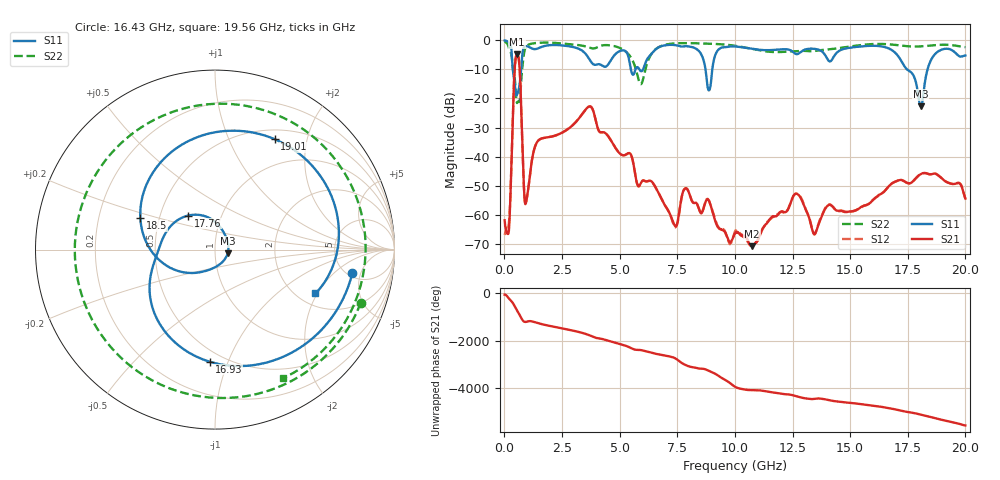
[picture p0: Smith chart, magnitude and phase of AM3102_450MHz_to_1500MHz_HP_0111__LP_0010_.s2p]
!Agilent Technologies,E8364B,MY43040894,A.07.50.67
!Agilent E8364B: A.07.50.67
!Date: Thursday, January 11, 2018 05:51:23
!Correction: S11(Full 2 Port(1,2))
!S21(Full 2 Port(1,2))
!S12(Full 2 Port(1,2))
!S22(Full 2 Port(1,2))
!S2P File: Measurements: S11, S21, S12, S22:
# Hz S  dB  R 50
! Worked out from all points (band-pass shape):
!   1601 points, 10 MHz to 20 GHz, reference 50 ohm
!   highest |S21| = -4.89 dB at 547.2 MHz (marker M1); lowest = -70.8 dB at 10.74 GHz (marker M2)
!   |S21| within 3 dB of the highest: 466.6 MHz to 646 MHz (179.3 MHz wide, 32.2 % of centre)
!   lowest |S11| = -22.7 dB at 18.06 GHz (marker M3), VSWR 1.16, Z = 57.5 - j2.39 ohm
!   |S11| at or under -10 dB: 366.7 MHz to 727.4 MHz (360.6 MHz wide, 65.9 % of centre); 8.724 GHz to 9.02 GHz (295.9 MHz wide, 3.33 % of centre); 17.47 GHz to 18.36 GHz (890.2 MHz wide, 4.97 % of centre)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
!   |S22| runs from -21.6 to -0.4 dB; largest |S21 - S12| = 0.0011
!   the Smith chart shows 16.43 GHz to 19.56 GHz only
!   S11 on the Smith chart (normalised r, x): 16.43 GHz: 5.55, -3.61; 16.93 GHz: 0.42, -0.86; 17.76 GHz: 0.70, +0.28; 18.5 GHz: 0.39, +0.17; 19.01 GHz: 0.62, +1.49; 19.56 GHz: 2.47, -1.92
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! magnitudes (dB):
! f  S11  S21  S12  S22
! 10 MHz  -0.1  -61.9  -66.9  -0.4
! 197.4 MHz  -0.7  -65.4  -62.9  -2.7
! 547.2 MHz  -18.5  -4.9  -4.9  -21.6
! 947 MHz  -2.0  -55.5  -55.4  -2.1
! 1.434 GHz  -2.9  -34.8  -34.9  -0.9
! 3.346 GHz  -3.4  -25.7  -25.7  -1.8
! 5.92 GHz  -10.6  -49.1  -49.2  -15.1
! 6.682 GHz  -2.5  -52.4  -52.4  -2.4
! 8.881 GHz  -17.2  -55.3  -55.2  -1.2
! 10.01 GHz  -2.1  -66.4  -65.7  -1.9
! 10.74 GHz  -2.9  -70.8  -70.5  -3.0
! 12.64 GHz  -4.7  -52.7  -52.7  -3.7
! 13.34 GHz  -2.9  -64.7  -64.6  -3.8
! 16.43 GHz  -2.2  -52.4  -52.3  -1.3
! 16.68 GHz  -2.8  -50.2  -50.3  -1.4
! 16.93 GHz  -4.1  -48.7  -48.7  -1.6
! 17.76 GHz  -12.4  -48.2  -48.2  -2.1
! 18.06 GHz  -22.7  -46.0  -46.0  -2.1
! 18.5 GHz  -6.9  -46.1  -46.0  -1.8
! 19.01 GHz  -3.1  -47.7  -47.7  -1.5
! 19.56 GHz  -4.3  -49.3  -49.3  -1.8
! 20 GHz  -5.2  -54.4  -54.5  -2.4
